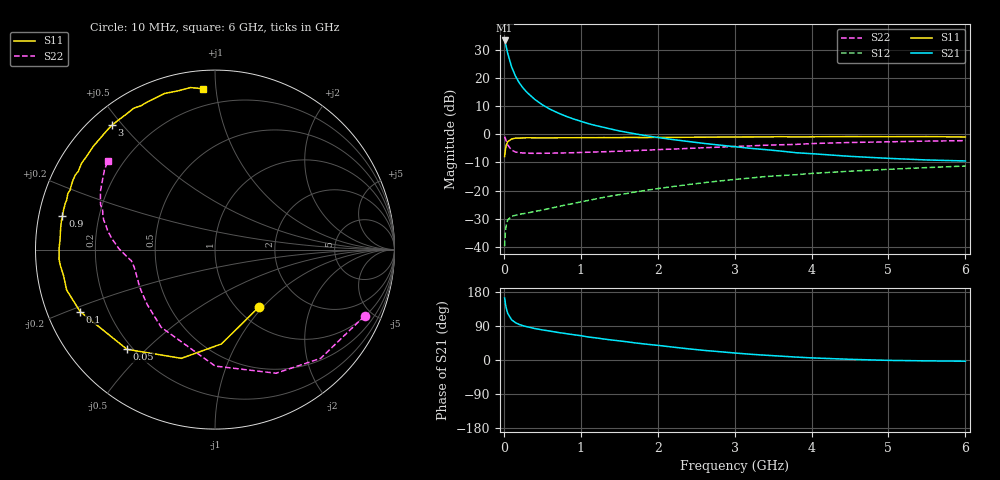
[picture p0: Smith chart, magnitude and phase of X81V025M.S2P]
! SIEMENS Small Signal Semiconductors
! BFP136W
! Si NPN RF Bipolar Junction Transistor in SOT343
! VCE = 1 V  IC = 25 mA
! Common Emitter S-Parameters:  September  1994
# GHz  S  MA  R  50
!  f  S11  S21  S12  S22
! GHz  MAG  ANG  MAG  ANG  MAG  ANG  MAG  ANG
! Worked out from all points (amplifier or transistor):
!   40 points, 10 MHz to 6 GHz, reference 50 ohm
!   highest |S21| = 33.5 dB at 10 MHz (marker M1)
!   |S21| within 3 dB of that: start of sweep to 37.61 MHz
!   unconditionally stable (mu >= 1): 738.7 MHz to 2.941 GHz; 5.862 GHz to end of sweep
!   at 200 MHz: K = 0.40, MSG = 23.4 dB, |S12| = -28.5 dB
!   at 1.5 GHz: K = 1.17, MAG = 8.9 dB, |S12| = -21.5 dB
!   at 6 GHz: K = 1.02, MAG = 0.1 dB, |S12| = -11.3 dB
!   S11 on the Smith chart (normalised r, x): 10 MHz: 1.24, -0.95; 50 MHz: 0.18, -0.44; 100 MHz: 0.10, -0.22; 900 MHz: 0.07, +0.11; 3 GHz: 0.06, +0.47; 6 GHz: 0.10, +0.92
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0.01  0.403 -52.8  47.08 163.7  0.0102 72.8  0.912 -23.9
0.02  0.5269 -86.1  42.17 149.4  0.018 60.1  0.8448 -45.8
0.03  0.6342 -107.2  37.17 138.1  0.0238 50.9  0.7684 -63.7
0.05  0.7409 -131.4  27.91 123.1  0.0299 37.6  0.6491 -89.9
0.1  0.8271 -155.3  16.05 106.3  0.0347 26.4  0.5266 -124.7
0.15  0.8567 -164.8  11.01 98.6  0.0362 23.9  0.4863 -140.8
0.2  0.856 -170.2  8.296 93.8  0.0377 24.2  0.4723 -149.8
0.25  0.8653 -173.8  6.701 90.4  0.0386 24.9  0.4664 -155.4
0.3  0.8706 -176.3  5.605 87.8  0.0396 25.9  0.4614 -159.3
0.4  0.8684 179.4  4.222 83.2  0.0423 30.2  0.4595 -164.1
0.5  0.865 176.2  3.366 79.4  0.0449 33.6  0.4604 -167.2
0.6  0.8666 173.9  2.809 76.3  0.0481 36.3  0.4628 -169.1
0.7  0.8694 171.0  2.422 72.8  0.0515 39.8  0.4651 -170.3
0.9  0.8704 167.5  1.893 66.9  0.0585 44.0  0.4713 -172.6
1.1  0.8731 162.8  1.552 60.7  0.0667 46.8  0.4808 -173.9
1.5  0.8766 156.1  1.153 50.5  0.0845 50.7  0.5014 -176.6
2.2  0.8845 143.5  0.807 34.0  0.1178 50.5  0.5469 177.8
3  0.9001 129.7  0.604 18.5  0.1574 45.8  0.6084 169.8
3.2  0.9003 126.3  0.565 15.3  0.1666 44.2  0.6229 167.5
4.5  0.9141 107.9  0.406 1.8  0.221 32.8  0.7164 153.0
5.5  0.9132 98.6  0.35 -2.3  0.256 24.7  0.7588 144.3
6  0.8987 94.3  0.336 -3.2  0.2731 20.2  0.7734 140.6
